(* Logix 5000 AddOnInstructionDefinition export CFW900_100150; software revision 20.06 *)

ADD_ON_INSTRUCTION CFW900_100150   (* revision 1.0, ExecutePrescan *)
// 100/150 WEG Advanced Speed
// AOI
// Help:
// Drive setup as follows:
// C9.2.1.1 - 3
// C9.2.1.2 - 7
// C9.2.1.3 - 5
// C9.2.1.4 - 60
// C9.2.1.5 - USER DEFINED
// C9.2.1.6 - USER DEFINED
// C9.2.1.7 - USER DEFINED
// C9.2.1.8 - USER DEFINED
// C9.2.2.2 - 100
// C9.2.2.3 - 101
// C9.2.2.4 - USER DEFINED
// C9.2.2.5 - USER DEFINED
// C9.2.2.6 - USER DEFINED
// C9.2.2.7 - USER DEFINED
// C9.2.2.8- USER DEFINED
// C9.5.1 = 100/150
// C9.5.2 = 1
// C9.5.3 = 8
// C9.5.4 = 1
// C9.5.5 = 8
// C4.1.1 - Ethernet
// C4.1.2 - Inactive
// C4.1.3 - Disable
// C4.2.2.1 - Ethernet
// C4.2.2.2 - Ethernet
// C4.2.2.3 - Ethernet
// C4.2.2.4 - Ethernet
// C4.3.1.2.1 - Keypad
// C4.3.1.2.2 - Ethernet
VAR_INPUT
   ConnectionFaulted : BOOL; {required}   // From CFW900
END_VAR
VAR_IN_OUT
   Inputs : INT[10]; {required}   // Input Assembly From CFW900
   Outputs : INT[10]; {required}   // Output Assembly To CFW900
END_VAR
VAR_INPUT
   cmd_DriveEnable : BOOL; {visible}   // 1 = Enable Operation of Drive 0 = Disable Operation of Drive
   cmd_NetCtrl : BOOL := 1; {visible}   // 1 = Remote (PLC) Control 0 = Local (HMI) Control
   cfg_RampSelect : BOOL; {visible}   // 1 = Ramp 2 (C6.1.4/C61.5) 0 = Ramp 1 (C6.1.1/C6.1.2)
   cmd_Fault_Reset : BOOL; {visible}   // 1 = Fault Reset 0 = No action
   cmd_QuickStop : BOOL := 1; {visible}   // 1 = NO Quick Stop 0 = Quick Stop
   cmd_RunForward : BOOL; {visible}   // 1 = Run Fwd 0 = Stop
   cmd_RunReverse : BOOL; {visible}   // 1 = Run Rev 0 = Stop
   cmd_JogForward : BOOL; {visible}   // 1 = Jog Fwd 0 = No Action / Stop
   cmd_JogReverse : BOOL; {visible}   // 1 = Jog Reverse 0 = No Action / Stop
   set_Speed_Reference : REAL; {required}   // Speed Setpoint (in %)
   cfg_FailToStartDelay : DINT; {access None, visible}
   cfg_FailToStopDelay : DINT; {access None, visible}
END_VAR
VAR_OUTPUT
   val_RealSpeed : REAL; {access Read Only, visible}   // Current Speed (in %)
   sts_Connection_Faulted : BOOL; {access Read Only, visible}   // Connection is interrupted status bit
   sts_Faulted : BOOL; {access Read Only, visible}   // 1 = Drive Faulted 0 = Drive not in Fault
   val_FaultCode : DINT; {access Read Only, visible}   // Fault Code 1 from Drive
   sts_Local : BOOL; {access Read Only, visible}   // 1 = Local 0 = Remote
   sts_Connection_Ready : BOOL; {access None, visible}   // Indicates that CFW900 connection is not in a faulted state
   sts_ConfigMode : BOOL; {access Read Only, visible}   // 1 = CFW900 in config mode 0 = CFW900 in operation mode
   sts_Ready : BOOL; {access Read Only, visible}   // 1 = Drive is ready to operate (states Ready, Enabled or Stopping) 0 = Drive is not ready to operate
   sts_STO : BOOL; {access Read Only, visible}   // 1 = Safe Torque Off (STO) Active 0 = STO Not Active
   sts_NoQuickStop : BOOL; {access Read Only, visible}   // 1 = No quick stop commanded 0 = Quick Stop commanded
   sts_Ctrl_from_net : BOOL; {access Read Only, visible}   // 1 = drive is controlled remotely (PLC) 0 = drive is controlled locally (HMI)
   sts_Ramp2_Selected : BOOL; {access None, visible}   // 1 = Ramp 2 rates selected 0 = Ramp 1 rates selected
   sts_RunCommand : BOOL; {access Read Only, visible}   // 1 = Commanded to run 0 = Not commanded to run
   sts_RunningForward : BOOL; {access Read Only, visible}   // 1 = CFW900 Running Forward 0 = CFW900 Stopped
   sts_RunningReverse : BOOL; {access Read Only, visible}   // 1 = CFW900 Running Reverse 0 = CFW900 not running reverse
   sts_FailedToStart : BOOL; {access Read Only, visible}   // Indicates Drive Failed to Start
   sts_FailedToStop : BOOL; {access None, visible}   // Indicates Drive Failed to stop in the time allotted
   val_OutputCurrent : REAL; {access Read Only, visible}   // Output current from Drive to Motor
   val_OutputFreq : REAL; {access Read Only, visible}   // Output Frequency in Hz
   val_OutputVoltage : DINT; {access Read Only, visible}   // Voltage Applied to Motor
END_VAR
VAR_INPUT
   set_Accel : REAL := 10.0; {required}   // Acceleration Ramp time (in seconds)
   set_Decel : REAL := 10.0; {required}   // Deceleration Ramp setpoint (0.1-999.9) in seconds
END_VAR
VAR_OUTPUT
   sts_STO_Fault : BOOL; {access Read Only, visible}   // STO has been tripped while run cmd active
END_VAR
VAR
   FailToStart : TIMER; {access None}
   Wrk_Run1 : BOOL; {access None}   // Internal bit to signal run1
   Wrk_Run2 : BOOL; {access None}   // Internal bit to signal run2
   FailToStop : TIMER; {access None}
   Wrk_Jog2 : BOOL; {access None}   // Internal bit for reverse Jog
   Wrk_Jog1 : BOOL; {access None}   // Internal Bit for forward Jog
   TempReal : REAL; {access None}
   TempDINT : DINT; {access None}
END_VAR

ROUTINE Logic   (* ladder *)
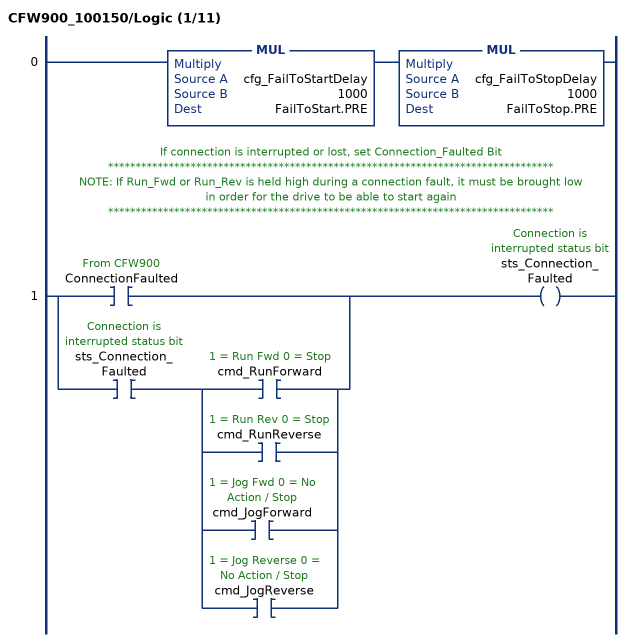
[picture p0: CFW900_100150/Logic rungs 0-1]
   0: MUL(cfg_FailToStartDelay,1000,FailToStart.PRE)MUL(cfg_FailToStopDelay,1000,FailToStop.PRE);
   // If connection is interrupted or lost, set Connection_Faulted Bit
   // *********************************************************************************
   // NOTE: If Run_Fwd or Run_Rev is held high during a connection fault, it must be brought low
   // in order for the drive to be able to start again
   // *********************************************************************************
   1: [XIC(ConnectionFaulted) ,XIC(sts_Connection_Faulted) [XIC(cmd_RunForward) ,XIC(cmd_RunReverse) ,XIC(cmd_JogForward) ,XIC(cmd_JogReverse) ] ]OTE(sts_Connection_Faulted);
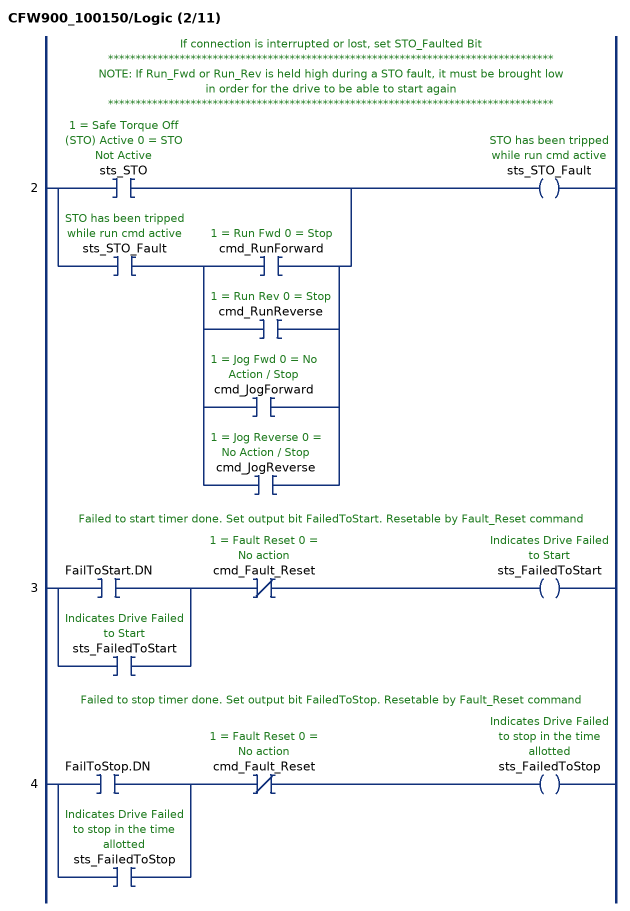
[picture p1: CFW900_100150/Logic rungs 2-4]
   // If connection is interrupted or lost, set STO_Faulted Bit
   // *********************************************************************************
   // NOTE: If Run_Fwd or Run_Rev is held high during a STO fault, it must be brought low
   // in order for the drive to be able to start again
   // *********************************************************************************
   2: [XIC(sts_STO) ,XIC(sts_STO_Fault) [XIC(cmd_RunForward) ,XIC(cmd_RunReverse) ,XIC(cmd_JogForward) ,XIC(cmd_JogReverse) ] ]OTE(sts_STO_Fault);
   // Failed to start timer done. Set output bit FailedToStart. Resetable by Fault_Reset command
   3: [XIC(FailToStart.DN) ,XIC(sts_FailedToStart) ]XIO(cmd_Fault_Reset)OTE(sts_FailedToStart);
   // Failed to stop timer done. Set output bit FailedToStop. Resetable by Fault_Reset command
   4: [XIC(FailToStop.DN) ,XIC(sts_FailedToStop) ]XIO(cmd_Fault_Reset)OTE(sts_FailedToStop);
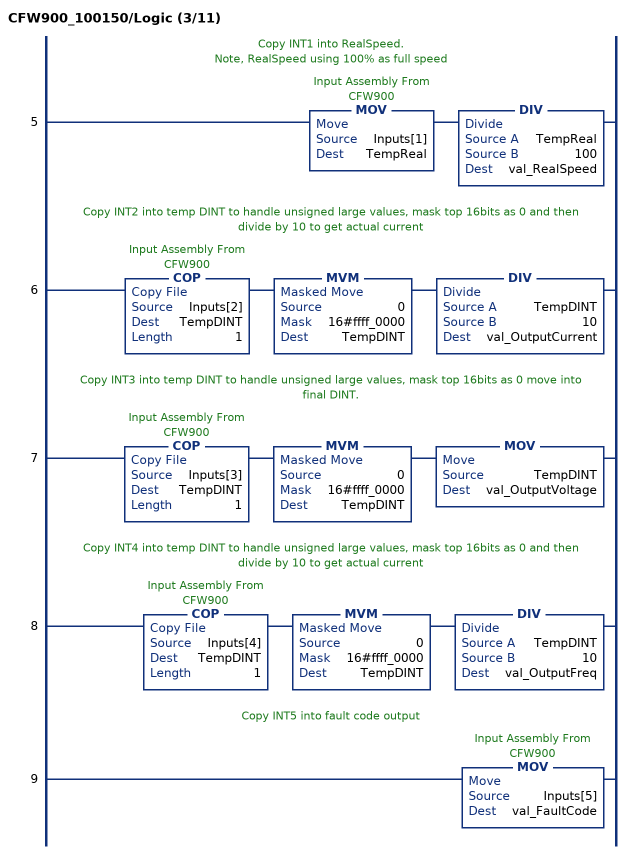
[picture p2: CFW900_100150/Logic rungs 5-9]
   // Copy INT1 into RealSpeed.
   // Note, RealSpeed using 100% as full speed
   5: MOV(Inputs[1],TempReal)DIV(TempReal,100,val_RealSpeed);
   // Copy INT2 into temp DINT to handle unsigned large values, mask top 16bits as 0 and then divide by 10 to get actual current
   6: COP(Inputs[2],TempDINT,1)MVM(0,16#ffff_0000,TempDINT)DIV(TempDINT,10,val_OutputCurrent);
   // Copy INT3 into temp DINT to handle unsigned large values, mask top 16bits as 0 move into final DINT.
   7: COP(Inputs[3],TempDINT,1)MVM(0,16#ffff_0000,TempDINT)MOV(TempDINT,val_OutputVoltage);
   // Copy INT4 into temp DINT to handle unsigned large values, mask top 16bits as 0 and then divide by 10 to get actual current
   8: COP(Inputs[4],TempDINT,1)MVM(0,16#ffff_0000,TempDINT)DIV(TempDINT,10,val_OutputFreq);
   // Copy INT5 into fault code output
   9: MOV(Inputs[5],val_FaultCode);
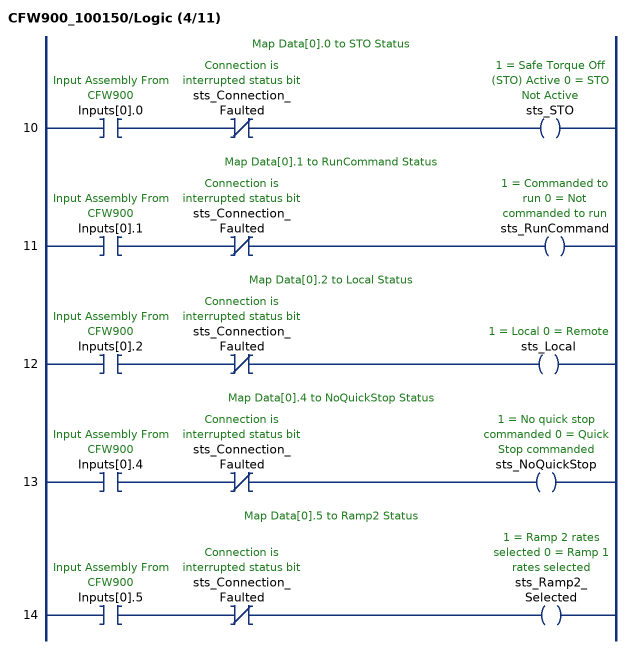
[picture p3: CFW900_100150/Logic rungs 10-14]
   // Map Data[0].0 to STO Status
   10: XIC(Inputs[0].0)XIO(sts_Connection_Faulted)OTE(sts_STO);
   // Map Data[0].1 to RunCommand Status
   11: XIC(Inputs[0].1)XIO(sts_Connection_Faulted)OTE(sts_RunCommand);
   // Map Data[0].2 to Local Status
   12: XIC(Inputs[0].2)XIO(sts_Connection_Faulted)OTE(sts_Local);
   // Map Data[0].4 to NoQuickStop Status
   13: XIC(Inputs[0].4)XIO(sts_Connection_Faulted)OTE(sts_NoQuickStop);
   // Map Data[0].5 to Ramp2 Status
   14: XIC(Inputs[0].5)XIO(sts_Connection_Faulted)OTE(sts_Ramp2_Selected);
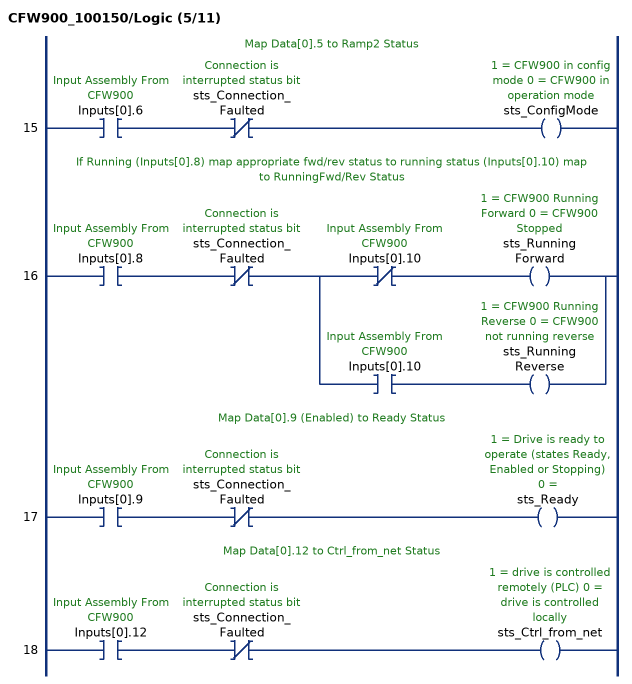
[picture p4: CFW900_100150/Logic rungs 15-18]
   // Map Data[0].5 to Ramp2 Status
   15: XIC(Inputs[0].6)XIO(sts_Connection_Faulted)OTE(sts_ConfigMode);
   // If Running (Inputs[0].8) map appropriate fwd/rev status to running status (Inputs[0].10) map to RunningFwd/Rev Status
   16: XIC(Inputs[0].8)XIO(sts_Connection_Faulted)[XIO(Inputs[0].10) OTE(sts_RunningForward) ,XIC(Inputs[0].10) OTE(sts_RunningReverse) ];
   // Map Data[0].9 (Enabled) to Ready Status
   17: XIC(Inputs[0].9)XIO(sts_Connection_Faulted)OTE(sts_Ready);
   // Map Data[0].12 to Ctrl_from_net Status
   18: XIC(Inputs[0].12)XIO(sts_Connection_Faulted)OTE(sts_Ctrl_from_net);
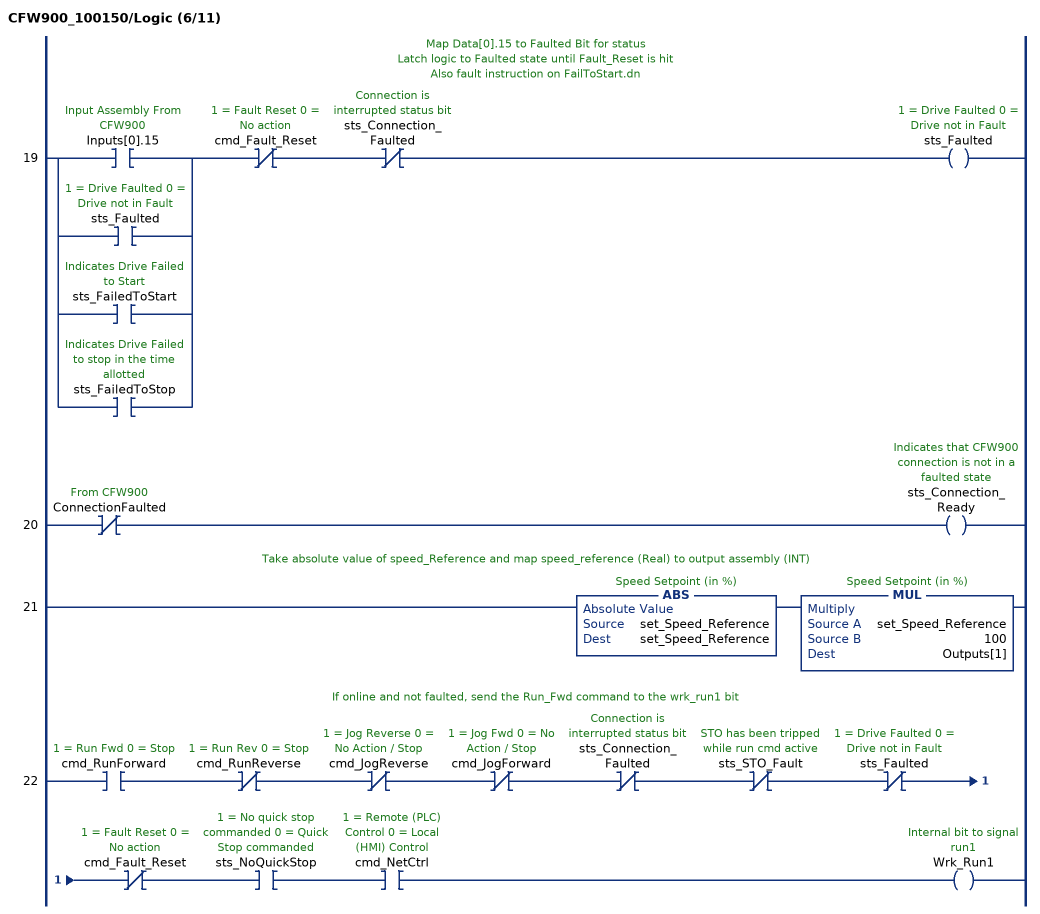
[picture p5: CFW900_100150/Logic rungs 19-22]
   // Map Data[0].15 to Faulted Bit for status
   // Latch logic to Faulted state until Fault_Reset is hit
   // Also fault instruction on FailToStart.dn
   19: [XIC(Inputs[0].15) ,XIC(sts_Faulted) ,XIC(sts_FailedToStart) ,XIC(sts_FailedToStop) ]XIO(cmd_Fault_Reset)XIO(sts_Connection_Faulted)OTE(sts_Faulted);
   20: XIO(ConnectionFaulted)OTE(sts_Connection_Ready);
   // Take absolute value of speed_Reference and map speed_reference (Real) to output assembly (INT)
   21: ABS(set_Speed_Reference,set_Speed_Reference)MUL(set_Speed_Reference,100,Outputs[1]);
   // If online and not faulted, send the Run_Fwd command to the wrk_run1 bit
   22: XIC(cmd_RunForward)XIO(cmd_RunReverse)XIO(cmd_JogReverse)XIO(cmd_JogForward)XIO(sts_Connection_Faulted)XIO(sts_STO_Fault)XIO(sts_Faulted)XIO(cmd_Fault_Reset)XIC(sts_NoQuickStop)XIC(cmd_NetCtrl)OTE(Wrk_Run1);
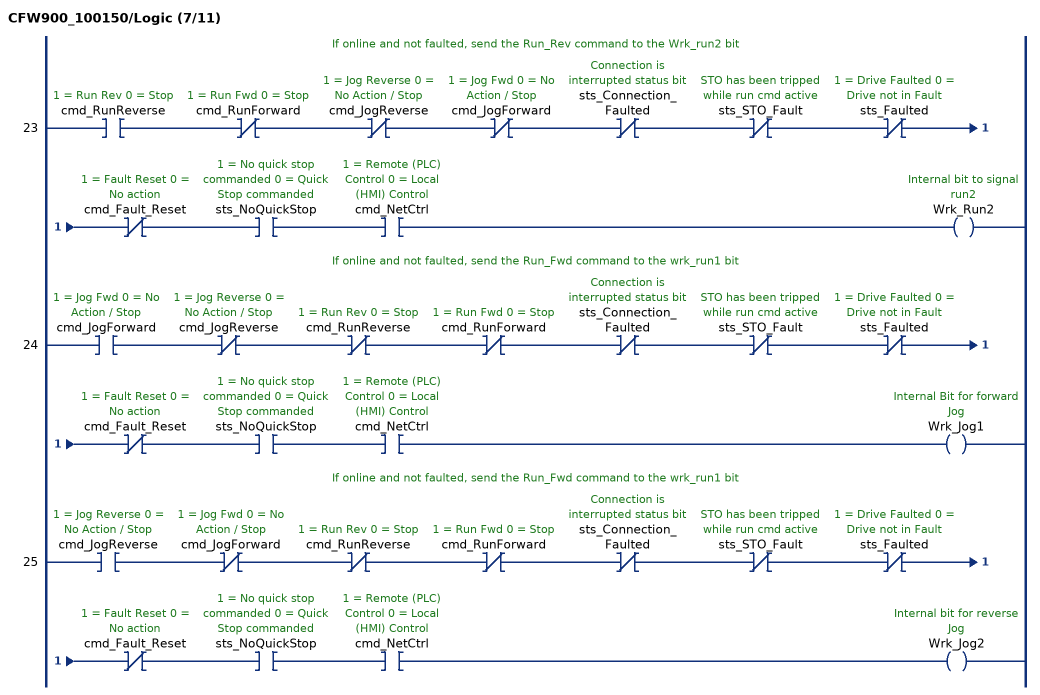
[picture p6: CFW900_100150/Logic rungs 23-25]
   // If online and not faulted, send the Run_Rev command to the Wrk_run2 bit
   23: XIC(cmd_RunReverse)XIO(cmd_RunForward)XIO(cmd_JogReverse)XIO(cmd_JogForward)XIO(sts_Connection_Faulted)XIO(sts_STO_Fault)XIO(sts_Faulted)XIO(cmd_Fault_Reset)XIC(sts_NoQuickStop)XIC(cmd_NetCtrl)OTE(Wrk_Run2);
   // If online and not faulted, send the Run_Fwd command to the wrk_run1 bit
   24: XIC(cmd_JogForward)XIO(cmd_JogReverse)XIO(cmd_RunReverse)XIO(cmd_RunForward)XIO(sts_Connection_Faulted)XIO(sts_STO_Fault)XIO(sts_Faulted)XIO(cmd_Fault_Reset)XIC(sts_NoQuickStop)XIC(cmd_NetCtrl)OTE(Wrk_Jog1);
   // If online and not faulted, send the Run_Fwd command to the wrk_run1 bit
   25: XIC(cmd_JogReverse)XIO(cmd_JogForward)XIO(cmd_RunReverse)XIO(cmd_RunForward)XIO(sts_Connection_Faulted)XIO(sts_STO_Fault)XIO(sts_Faulted)XIO(cmd_Fault_Reset)XIC(sts_NoQuickStop)XIC(cmd_NetCtrl)OTE(Wrk_Jog2);
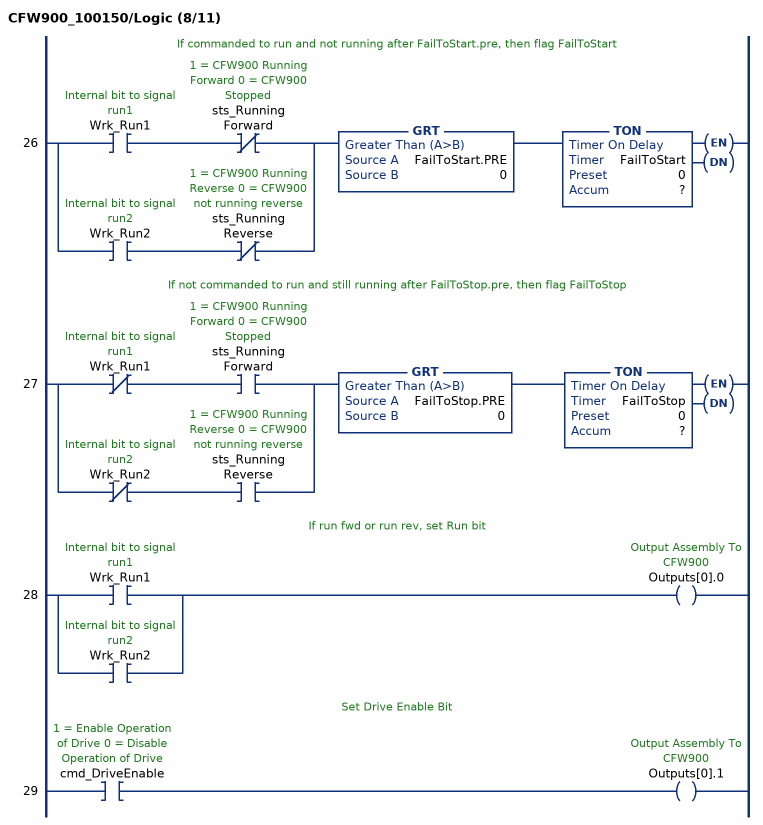
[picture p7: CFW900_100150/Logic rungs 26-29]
   // If commanded to run and not running after FailToStart.pre, then flag FailToStart
   26: [XIC(Wrk_Run1) XIO(sts_RunningForward) ,XIC(Wrk_Run2) XIO(sts_RunningReverse) ]GRT(FailToStart.PRE,0)TON(FailToStart,?,?);
   // If not commanded to run and still running after FailToStop.pre, then flag FailToStop
   27: [XIO(Wrk_Run1) XIC(sts_RunningForward) ,XIO(Wrk_Run2) XIC(sts_RunningReverse) ]GRT(FailToStop.PRE,0)TON(FailToStop,?,?);
   // If run fwd or run rev, set Run bit
   28: [XIC(Wrk_Run1) ,XIC(Wrk_Run2) ]OTE(Outputs[0].0);
   // Set Drive Enable Bit
   29: XIC(cmd_DriveEnable)OTE(Outputs[0].1);
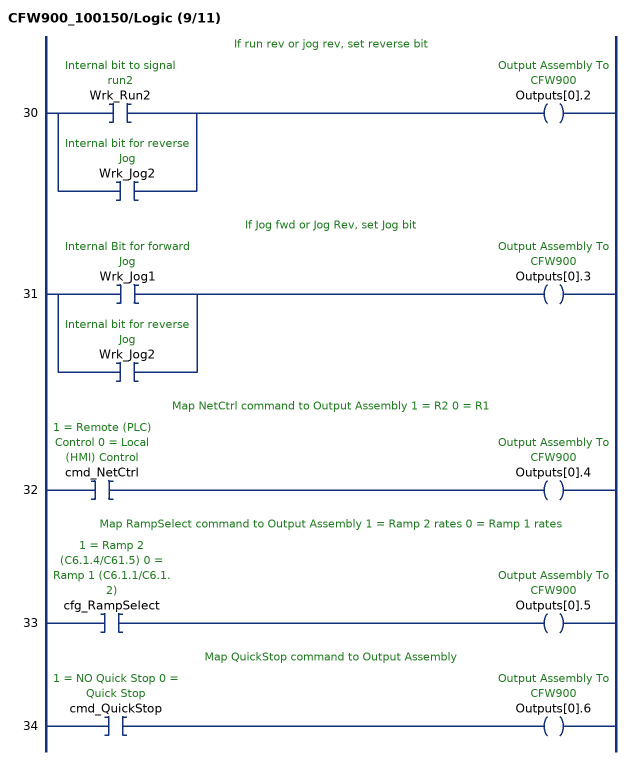
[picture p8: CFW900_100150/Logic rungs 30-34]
   // If run rev or jog rev, set reverse bit
   30: [XIC(Wrk_Run2) ,XIC(Wrk_Jog2) ]OTE(Outputs[0].2);
   // If Jog fwd or Jog Rev, set Jog bit
   31: [XIC(Wrk_Jog1) ,XIC(Wrk_Jog2) ]OTE(Outputs[0].3);
   // Map NetCtrl command to Output Assembly 1 = R2 0 = R1
   32: XIC(cmd_NetCtrl)OTE(Outputs[0].4);
   // Map RampSelect command to Output Assembly 1 = Ramp 2 rates 0 = Ramp 1 rates
   33: XIC(cfg_RampSelect)OTE(Outputs[0].5);
   // Map QuickStop command to Output Assembly
   34: XIC(cmd_QuickStop)OTE(Outputs[0].6);
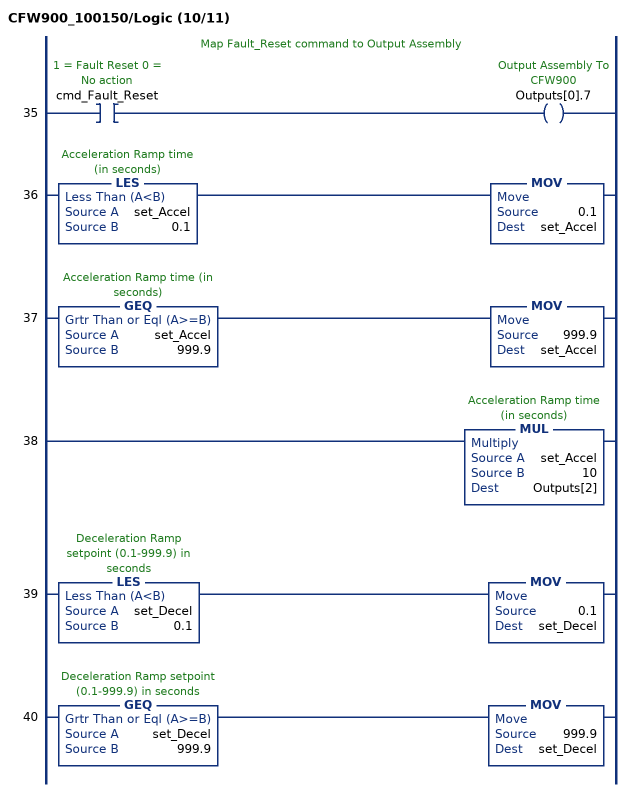
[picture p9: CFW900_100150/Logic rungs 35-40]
   // Map Fault_Reset command to Output Assembly
   35: XIC(cmd_Fault_Reset)OTE(Outputs[0].7);
   36: LES(set_Accel,0.1)MOV(0.1,set_Accel);
   37: GEQ(set_Accel,999.9)MOV(999.9,set_Accel);
   38: MUL(set_Accel,10,Outputs[2]);
   39: LES(set_Decel,0.1)MOV(0.1,set_Decel);
   40: GEQ(set_Decel,999.9)MOV(999.9,set_Decel);
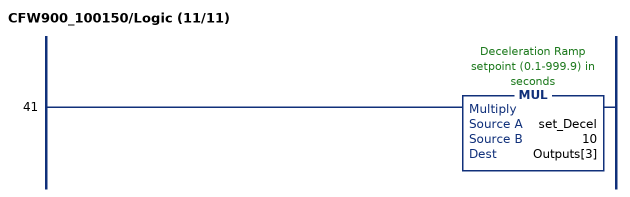
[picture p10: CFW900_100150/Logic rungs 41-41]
   41: MUL(set_Decel,10,Outputs[3]);
END_ROUTINE

ROUTINE Prescan   (* ladder *)
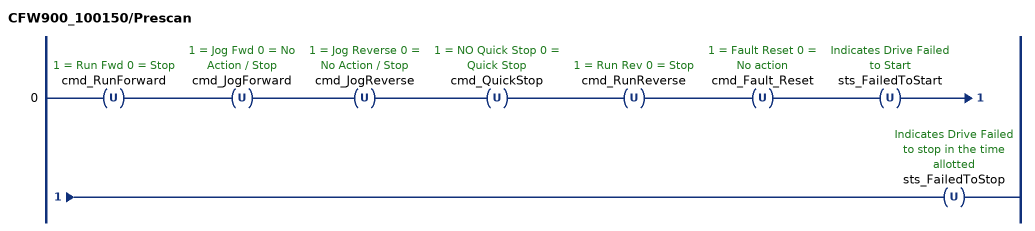
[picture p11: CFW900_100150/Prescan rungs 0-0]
   0: OTU(cmd_RunForward)OTU(cmd_JogForward)OTU(cmd_JogReverse)OTU(cmd_QuickStop)OTU(cmd_RunReverse)OTU(cmd_Fault_Reset)OTU(sts_FailedToStart)OTU(sts_FailedToStop);
END_ROUTINE
END_ADD_ON_INSTRUCTION
